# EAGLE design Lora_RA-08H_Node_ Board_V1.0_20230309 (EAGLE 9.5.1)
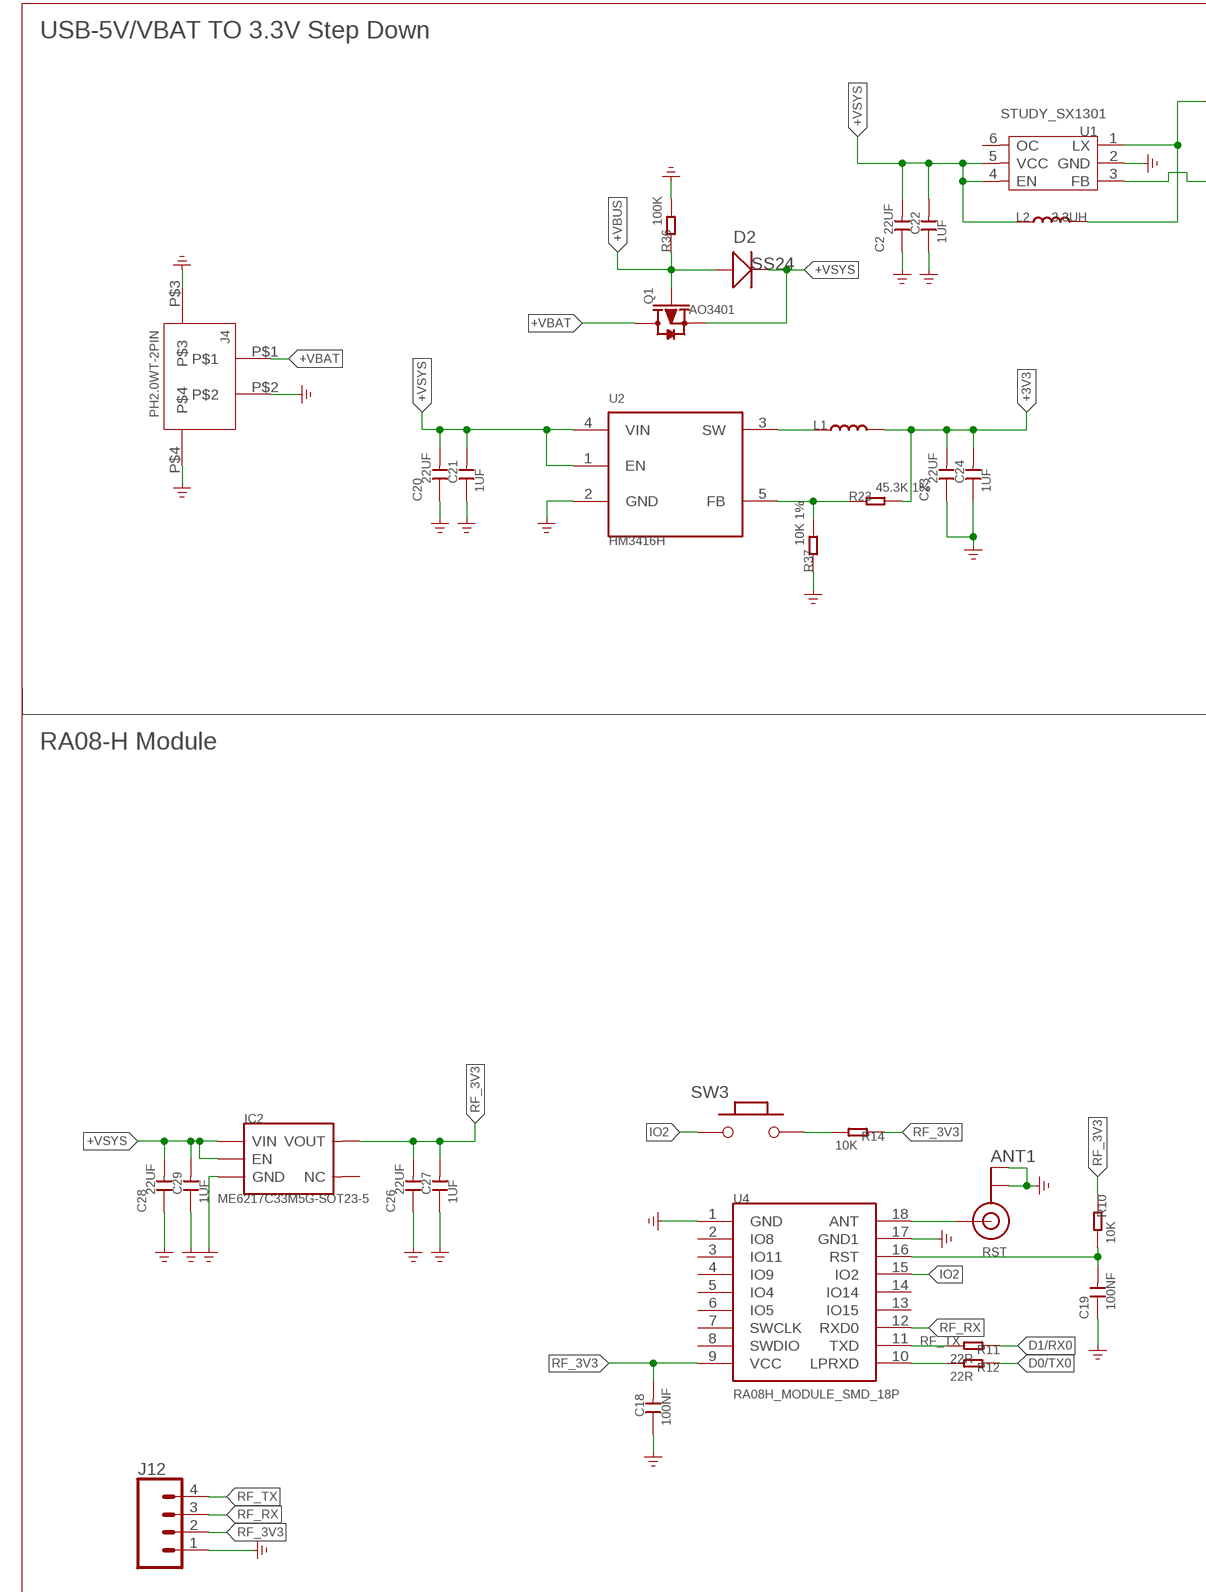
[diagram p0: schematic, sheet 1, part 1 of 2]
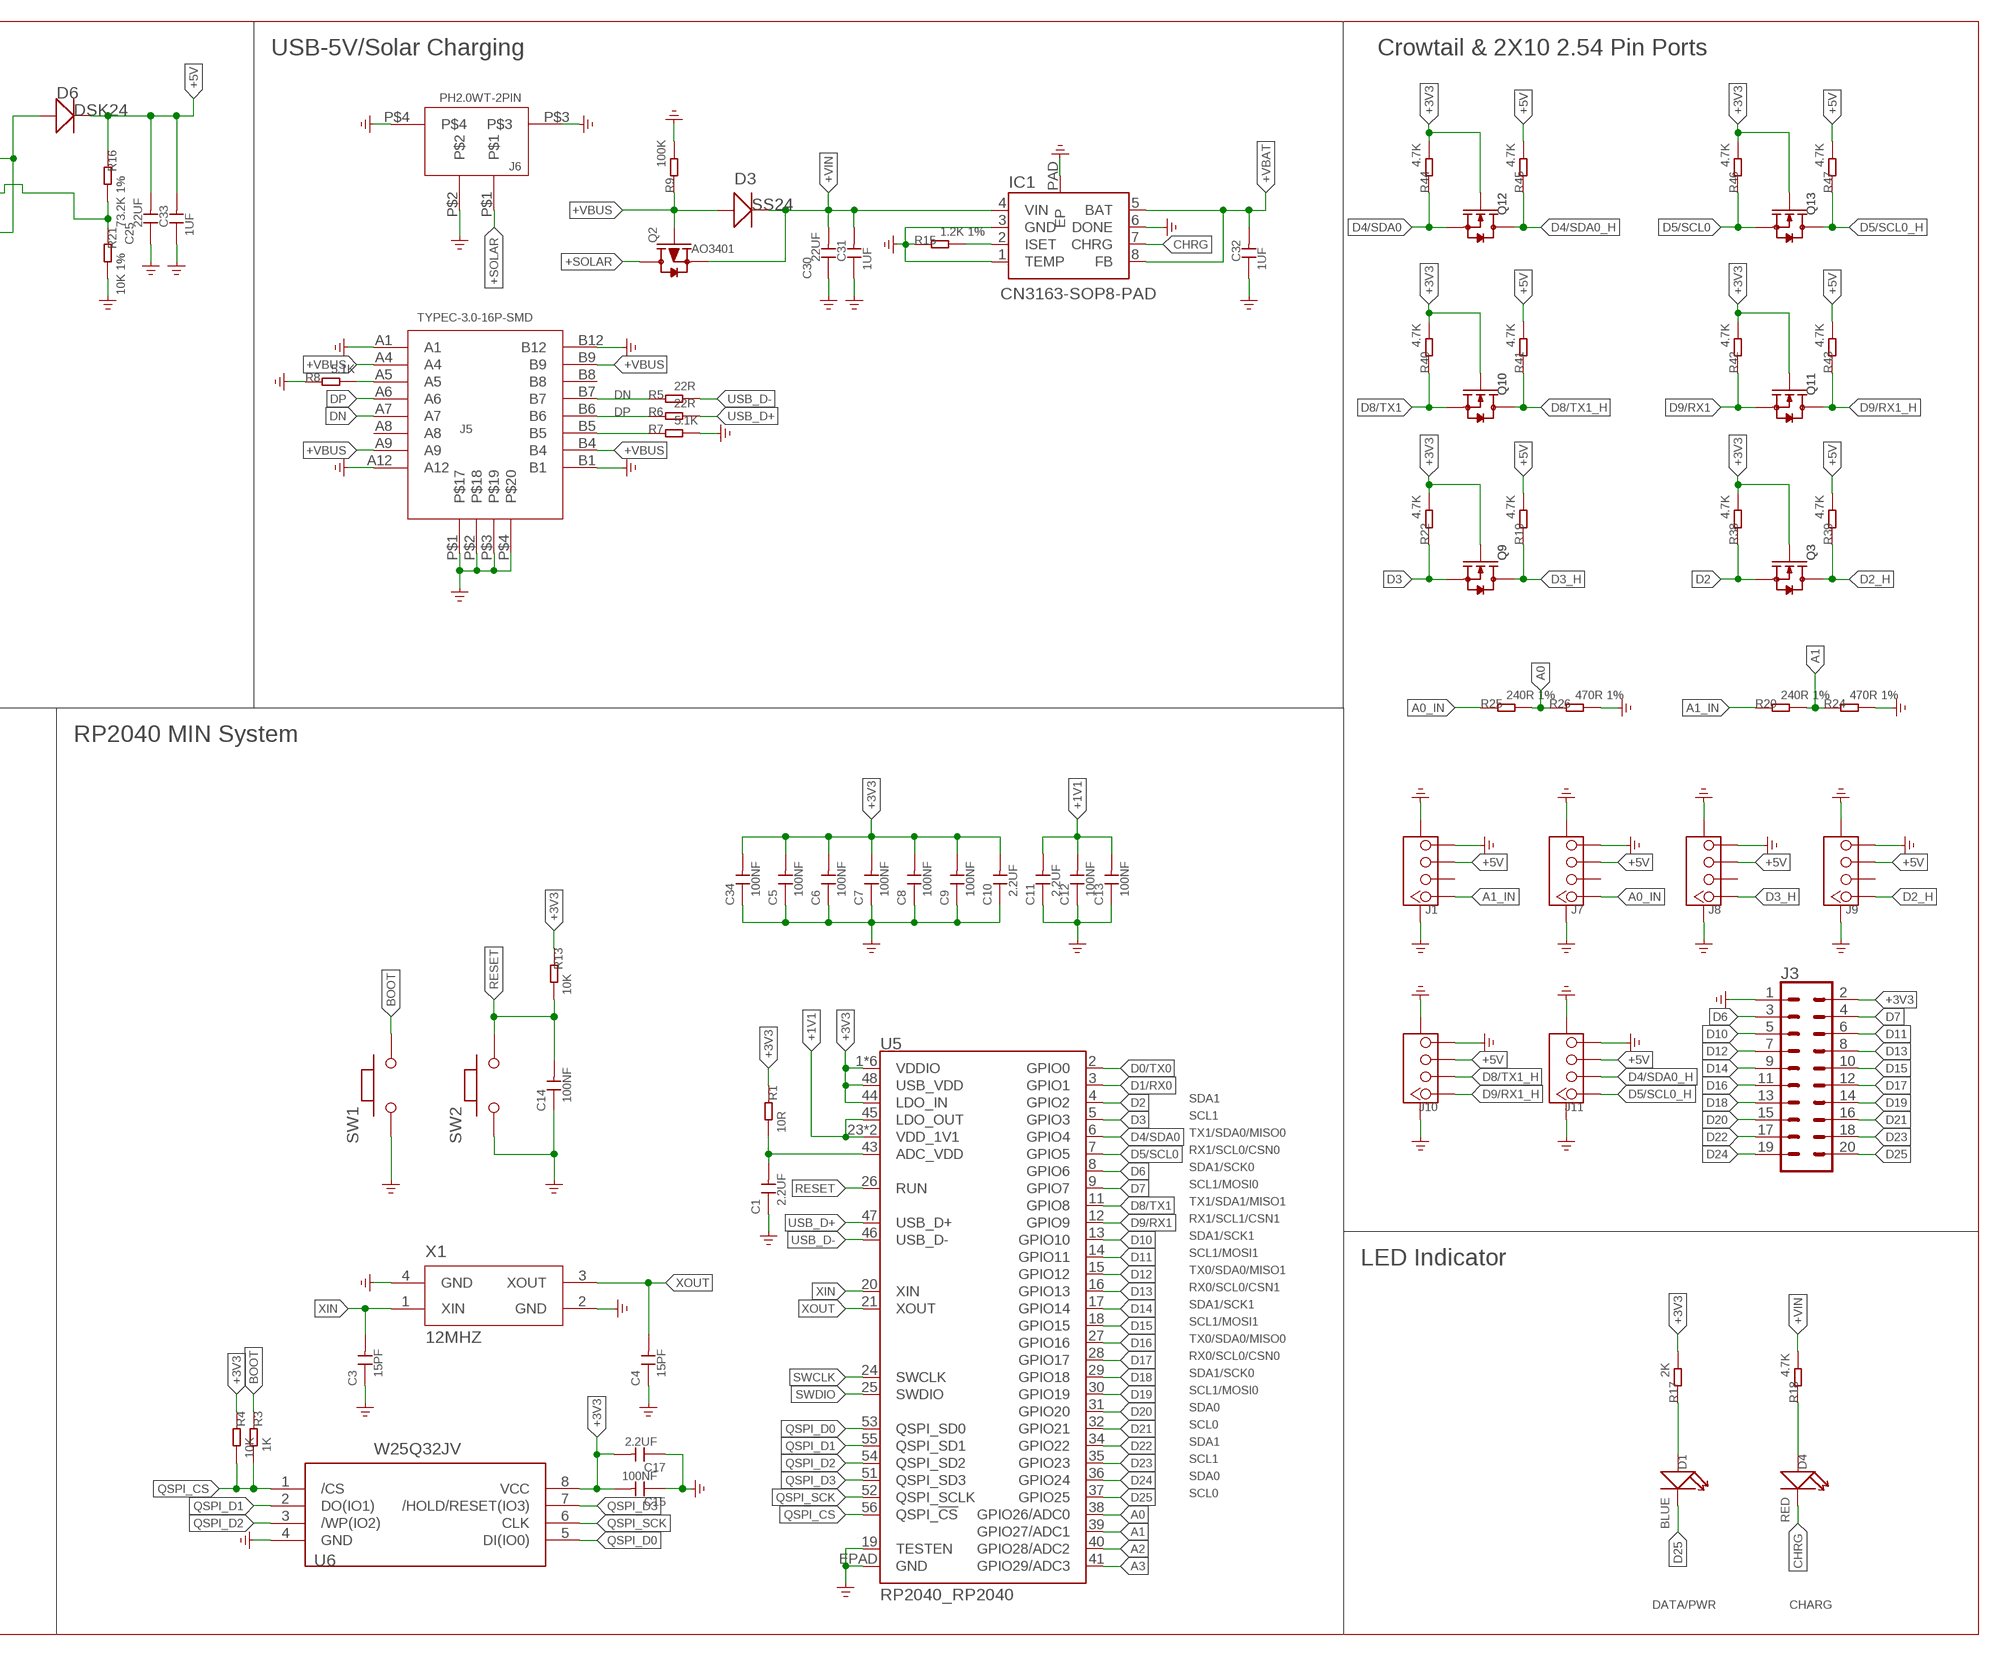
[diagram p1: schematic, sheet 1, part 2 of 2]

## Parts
ANT1  SPARKFUN2_U.FL  [SPARKFUN2_U.FL]
C1  2.2UF  CAPC0402-1  [0402]
C2  22UF  C0805  [C0805]
C3  15PF  CAPC0402-1  [0402]
C4  15PF  CAPC0402-1  [0402]
C5  100NF  CAPC0402-1  [0402]
C6  100NF  CAPC0402-1  [0402]
C7  100NF  CAPC0402-1  [0402]
C8  100NF  CAPC0402-1  [0402]
C9  100NF  CAPC0402-1  [0402]
C10  2.2UF  CAPC0402-1  [0402]
C11  2.2UF  CAPC0402-1  [0402]
C12  100NF  CAPC0402-1  [0402]
C13  100NF  CAPC0402-1  [0402]
C14  100NF  CAPC0402-1  [0402]
C15  100NF  CAPC0402-1  [0402]
C17  2.2UF  CAPC0402-1  [0402]
C18  100NF  C0603  [C0603]
C19  100NF  CAPC0402-1  [0402]
C20  22UF  C0805  [C0805]
C21  1UF  C0603  [C0603]
C22  1UF  C0603  [C0603]
C23  22UF  C0805  [C0805]
C24  1UF  C0603  [C0603]
C25  22UF  C0805  [C0805]
C26  22UF  C0805  [C0805]
C27  1UF  C0603  [C0603]
C28  22UF  C0805  [C0805]
C29  1UF  C0603  [C0603]
C30  22UF  C0805  [C0805]
C31  1UF  C0603  [C0603]
C32  1UF  C0603  [C0603]
C33  1UF  C0603  [C0603]
C34  100NF  CAPC0402-1  [0402]
D1  BLUE  LED-SMT0603  [LED0603]
D2  SS24  DIODEB130L-13-F  [SMA]
D3  SS24  DIODEB130L-13-F  [SMA]
D4  RED  LED-SMT0603  [LED0603]
D6  DSK24  DIODE  [D_SOD123FL]
IC1  CN3163-SOP8-PAD  [SOP8-PAD]
IC2  ME6217C33M5G-SOT23-5  [IC_SOT23-5]
J1  CONNECTOR_TWIG-4P-2.0-SMD-FEMALE-REINFORCE90D  [CONNECTOR_4P-SMD-2.0-90D]
J3  CONN_10X22X10-DSY-P2.54  [2X10-DSY-P2.54]
J4  PH2.0WT-2PIN  [PH2.0WT-2PIN]
J5  TYPEC-3.0-16P-SMD  [KEVIN_3.0TYPEC-SMD]
J6  PH2.0WT-2PIN  [PH2.0WT-2PIN]
J7  CONNECTOR_TWIG-4P-2.0-SMD-FEMALE-REINFORCE90D  [CONNECTOR_4P-SMD-2.0-90D]
J8  CONNECTOR_TWIG-4P-2.0-SMD-FEMALE-REINFORCE90D  [CONNECTOR_4P-SMD-2.0-90D]
J9  CONNECTOR_TWIG-4P-2.0-SMD-FEMALE-REINFORCE90D  [CONNECTOR_4P-SMD-2.0-90D]
J10  CONNECTOR_TWIG-4P-2.0-SMD-FEMALE-REINFORCE90D  [CONNECTOR_4P-SMD-2.0-90D]
J11  CONNECTOR_TWIG-4P-2.0-SMD-FEMALE-REINFORCE90D  [CONNECTOR_4P-SMD-2.0-90D]
J12  CONN_041.27MM  [1X04_1.27MM]
L1  LL0420  [L0420]
L2  3.3UH  LL0420  [L0420]
Q1  AO3401  MOSFET-PSOT23  [PMOS_SOT23]
Q2  AO3401  MOSFET-PSOT23  [PMOS_SOT23]
Q3  MOSFET-NSI1304BDL  [MOS_SOT323]
Q9  MOSFET-NSI1304BDL  [MOS_SOT323]
Q10  MOSFET-NSI1304BDL  [MOS_SOT323]
Q11  MOSFET-NSI1304BDL  [MOS_SOT323]
Q12  MOSFET-NSI1304BDL  [MOS_SOT323]
Q13  MOSFET-NSI1304BDL  [MOS_SOT323]
R1  10R  RES-0402  [R0402]
R3  1K  RES-0402  [R0402]
R4  10K  RES-0402  [R0402]
R5  22R  RES-0402  [R0402]
R6  22R  RES-0402  [R0402]
R7  5.1K  RES-0402  [R0402]
R8  5.1K  RES-0402  [R0402]
R9  100K  RES-0402  [R0402]
R10  10K  RES-0402  [R0402]
R11  22R  RES-0402  [R0402]
R12  22R  RES-0402  [R0402]
R13  10K  RES-0402  [R0402]
R14  10K  RES-0402  [R0402]
R15  1.2K 1%  RES-0402  [R0402]
R16  73.2K 1%  RES-0402  [R0402]
R17  2K  RES-0402  [R0402]
R18  4.7K  RES-0402  [R0402]
R19  4.7K  RES-0402  [R0402]
R20  240R 1%  RES-0402  [R0402]
R21  10K 1%  RES-0402  [R0402]
R22  4.7K  RES-0402  [R0402]
R23  45.3K 1%  RES-0402  [R0402]
R24  470R 1%  RES-0402  [R0402]
R25  240R 1%  RES-0402  [R0402]
R26  470R 1%  RES-0402  [R0402]
R36  100K  RES-0402  [R0402]
R37  10K 1%  RES-0402  [R0402]
R38  4.7K  RES-0402  [R0402]
R39  4.7K  RES-0402  [R0402]
R40  4.7K  RES-0402  [R0402]
R41  4.7K  RES-0402  [R0402]
R42  4.7K  RES-0402  [R0402]
R43  4.7K  RES-0402  [R0402]
R44  4.7K  RES-0402  [R0402]
R45  4.7K  RES-0402  [R0402]
R46  4.7K  RES-0402  [R0402]
R47  4.7K  RES-0402  [R0402]
SW1  MYSMD_PB157_4.3X3  [MYSMD_157SW]
SW2  MYSMD_PB157_4.3X3  [MYSMD_157SW]
SW3  MYSMD_PB157_4.3X3  [MYSMD_157SW]
U1  STUDY_SX1301  [STUDY_SOT23-6L]
U2  HM3416H  [IC_SOT23-5]
U4  RA08H_MODULE_SMD_18P  [RA08H_MODULE_SMT_18P]
U5  RP2040_RP2040  [RP2040_QFN-56]
U6  W25Q32JV  [SELF_SOIC-8-208MIL]
X1  12MHZ  XTAL-SMD3225  [SMD3225]

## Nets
+1V1: C11.2 C12.2 C13.2 U5.23(VDD_1V1) U5.45(LDO_OUT) U5.50(VDD_1V1)
+3V3: C5.2 C6.2 C7.2 C8.2 C9.2 C10.2 C15.2 C17.2 C23.2 C24.2 C34.2 J3.2 L1.2 Q3.1(G) Q9.1(G) Q10.1(G) Q11.1(G) Q12.1(G) Q13.1(G) R1.1 R4.1 R13.1 R17.2 R22.2 R23.2 R38.2 R40.2 R42.2 R44.2 R46.2 U5.1(VDDIO) U5.10(VDDIO) U5.22(VDDIO) U5.33(VDDIO) U5.42(VDDIO) U5.44(LDO_IN) U5.48(USB_VDD) U5.49(VDDIO) U6.8(VCC)
+5V: C25.2 C33.2 D6.- J1.3 J7.3 J8.3 J9.3 J10.3 J11.3 R16.1 R19.2 R39.2 R41.2 R43.2 R45.2 R47.2
+SOLAR: J6.P$1 Q2.3(D)
+VBAT: C32.2 IC1.5(BAT) IC1.8(FB) J4.P$1 Q1.3(D)
+VBUS: D2.2(+) D3.2(+) J5.A4 J5.A9 J5.B4 J5.B9 Q1.1(G) Q2.1(G) R9.1 R36.1
+VIN: C30.2 C31.2 D3.1(-) IC1.4(VIN) Q2.2(S) R18.2
+VSYS: C2.2 C20.2 C21.2 C22.2 C28.2 C29.2 D2.1(-) IC2.1(VIN) IC2.3(EN) L2.1 Q1.2(S) U1.4(EN) U1.5(VCC) U2.1(EN) U2.4(VIN)
A0: R25.2 R26.1 U5.38(GPIO26/ADC0)
A0_IN: J7.1 R25.1
A1: R20.2 R24.1 U5.39(GPIO27/ADC1)
A1_IN: J1.1 R20.1
A2: U5.40(GPIO28/ADC2)
A3: U5.41(GPIO29/ADC3)
BOOT: R3.1 SW1.2
CHRG: D4.- IC1.7(CHRG)
D0/TX0: R12.1 U5.2(GPIO0)
D1/RX0: R11.1 U5.3(GPIO1)
D2: Q3.2(S) R38.1 U5.4(GPIO2)
D2_H: J9.1 Q3.3(D) R39.1
D3: Q9.2(S) R22.1 U5.5(GPIO3)
D3_H: J8.1 Q9.3(D) R19.1
D4/SDA0: Q12.2(S) R44.1 U5.6(GPIO4)
D4/SDA0_H: J11.2 Q12.3(D) R45.1
D5/SCL0: Q13.2(S) R46.1 U5.7(GPIO5)
D5/SCL0_H: J11.1 Q13.3(D) R47.1
D6: J3.3 U5.8(GPIO6)
D7: J3.4 U5.9(GPIO7)
D8/TX1: Q10.2(S) R40.1 U5.11(GPIO8)
D8/TX1_H: J10.2 Q10.3(D) R41.1
D9/RX1: Q11.2(S) R42.1 U5.12(GPIO9)
D9/RX1_H: J10.1 Q11.3(D) R43.1
D10: J3.5 U5.13(GPIO10)
D11: J3.6 U5.14(GPIO11)
D12: J3.7 U5.15(GPIO12)
D13: J3.8 U5.16(GPIO13)
D14: J3.9 U5.17(GPIO14)
D15: J3.10 U5.18(GPIO15)
D16: J3.11 U5.27(GPIO16)
D17: J3.12 U5.28(GPIO17)
D18: J3.13 U5.29(GPIO18)
D19: J3.14 U5.30(GPIO19)
D20: J3.15 U5.31(GPIO20)
D21: J3.16 U5.32(GPIO21)
D22: J3.17 U5.34(GPIO22)
D23: J3.18 U5.35(GPIO23)
D24: J3.19 U5.36(GPIO24)
D25: D1.- J3.20 U5.37(GPIO25)
DN: J5.A7 J5.B7 R5.1
DP: J5.A6 J5.B6 R6.1
GND: ANT1.P$1(GND) ANT1.P$2(GND) C1.1 C2.1 C3.1 C4.1 C5.1 C6.1 C7.1 C8.1 C9.1 C10.1 C11.1 C12.1 C13.1 C14.1 C15.1 C17.1 C18.1 C19.1 C20.1 C21.1 C22.1 C23.1 C24.1 C25.1 C26.1 C27.1 C28.1 C29.1 C30.1 C31.1 C32.1 C33.1 C34.1 IC1.1(TEMP) IC1.3(GND) IC1.6(DONE) IC1.PAD(EP) IC2.2(GND) J1.4 J1.SS1 J1.SS2 J3.1 J4.P$2 J4.P$3 J4.P$4 J5.A1 J5.A12 J5.B1 J5.B12 J5.P$1 J5.P$2 J5.P$3 J5.P$4 J6.P$2 J6.P$3 J6.P$4 J7.4 J7.SS1 J7.SS2 J8.4 J8.SS1 J8.SS2 J9.4 J9.SS1 J9.SS2 J10.4 J10.SS1 J10.SS2 J11.4 J11.SS1 J11.SS2 J12.1 R7.2 R8.1 R9.2 R15.1 R21.2 R24.2 R26.2 R36.2 R37.1 SW1.1 SW2.1 U1.2(GND) U2.2(GND) U4.1(GND) U4.17(GND1) U5.19(TESTEN) U5.EPAD(GND) U6.4(GND) X1.2(GND) X1.4(GND)
IO2: SW3.1 U4.15(IO2)
N$1: C1.2 R1.2 U5.43(ADC_VDD)
N$2: J5.B5 R7.1
N$3: L1.1 U2.3(SW)
N$4: D6.+ L2.2 U1.1(LX)
N$5: R12.2 U4.10(LPRXD)
N$6: J5.A5 R8.2
N$7: R14.2 SW3.2
N$8: ANT1.P$3(SIGNAL) U4.18(ANT)
N$9: R23.1 R37.2 U2.5(FB)
N$10: IC1.2(ISET) R15.2
N$11: D4.+ R18.1
N$13: R16.2 R21.1 U1.3(FB)
N$14: D1.+ R17.1
QSPI_CS: R3.2 R4.2 U5.56(QSPI_!CS!) U6.1(/CS)
QSPI_D0: U5.53(QSPI_SD0) U6.5(DI(IO0))
QSPI_D1: U5.55(QSPI_SD1) U6.2(DO(IO1))
QSPI_D2: U5.54(QSPI_SD2) U6.3(/WP(IO2))
QSPI_D3: U5.51(QSPI_SD3) U6.7(/HOLD/RESET(IO3))
QSPI_SCK: U5.52(QSPI_SCLK) U6.6(CLK)
RESET: C14.2 R13.2 SW2.2 U5.26(RUN)
RF_3V3: C18.2 C26.2 C27.2 IC2.5(VOUT) J12.2 R10.1 R14.1 U4.9(VCC)
RF_RX: J12.3 U4.12(RXD0)
RF_TX: J12.4 R11.2 U4.11(TXD)
RST: C19.2 R10.2 U4.16(RST)
SWCLK: U5.24(SWCLK)
SWDIO: U5.25(SWDIO)
USB_D+: R6.2 U5.47(USB_D+)
USB_D-: R5.2 U5.46(USB_D-)
XIN: C3.2 U5.20(XIN) X1.1(XIN)
XOUT: C4.2 U5.21(XOUT) X1.3(XOUT)
Unconnected: IC2.4(NC) J1.2 J5.A8 J5.B8 J7.2 J8.2 J9.2 U1.6(OC) U4.2(IO8) U4.3(IO11) U4.4(IO9) U4.5(IO4) U4.6(IO5) U4.7(SWCLK) U4.8(SWDIO) U4.13(IO15) U4.14(IO14)

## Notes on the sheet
- USB-5V/VBAT TO 3.3V Step Down | USB-5V/Solar Charging | Crowtail & 2X10 2.54 Pin Ports
- RA08-H Module | RP2040 MIN System
- SDA1
- SCL1
- TX1/SDA0/MISO0
- RX1/SCL0/CSN0
- SDA1/SCK0
- SCL1/MOSI0
- TX1/SDA1/MISO1
- RX1/SCL1/CSN1
- SDA1/SCK1
- SCL1/MOSI1
- LED Indicator
- TX0/SDA0/MISO1
- RX0/SCL0/CSN1
- SDA1/SCK1
- SCL1/MOSI1
- TX0/SDA0/MISO0
- RX0/SCL0/CSN0
- SDA1/SCK0
- SCL1/MOSI0
- SDA0
- SCL0
- SDA1
- SCL1
- SDA0
- SCL0
- DATA/PWR | CHARG

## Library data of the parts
ANT1 = Lora_RA-08H_Node_ Board:SPARKFUN2_U.FL
C1 C3-C15 C17 C19 C34 = Lora_RA-08H_Node_ Board:CAP*
C2 C20 C23 C25 C26 C28 C30 = Lora_RA-08H_Node_ Board:C0805
C18 C21 C22 C24 C27 C29 C31-C33 = Lora_RA-08H_Node_ Board:C0603
D1 D4 = Lora_RA-08H_Node_ Board:LED-SMT*
D2 D3 D6 = Lora_RA-08H_Node_ Board:DIODE*
IC1 = Lora_RA-08H_Node_ Board:CN3163-SOP8-PAD
IC2 = Lora_RA-08H_Node_ Board:ME6217C33M5G-SOT23-5
J1 J7-J11 = Lora_RA-08H_Node_ Board:CONNECTOR_TWIG-4P-2.0-SMD-FEMALE-REINFORCE
J3 = Lora_RA-08H_Node_ Board:CONN_10X2: Multi connection point. Often used as Generic Header-pin footprint for 0.1 inch spaced/style header connections On any of the 0.1 inch spaced packages, you can populate with these: Break Away Headers - Straight (PRT-00116) Break Away Male Headers - Right Angle (PRT-00553) Female Headers (PRT-00115)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
J4 J6 = Lora_RA-08H_Node_ Board:PH2.0WT-2PIN
J5 = Lora_RA-08H_Node_ Board:TYPEC-3.0-16P-SMD
J12 = Lora_RA-08H_Node_ Board:CONN_04: Multi connection point. Often used as Generic Header-pin footprint for 0.1 inch spaced/style header connections On any of the 0.1 inch spaced packages, you can populate with these: Break Away Headers - Straight (PRT-00116) Break Away Male Headers - Right Angle (PRT-00553) Female Headers (PRT-00115)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
L1 L2 = Lora_RA-08H_Node_ Board:L*
Q1 Q2 = Lora_RA-08H_Node_ Board:MOSFET-P: IRLL014: http://www.vishay.com/docs/91319/sihll014.pdf
Q3 Q9-Q13 = Lora_RA-08H_Node_ Board:MOSFET-N*: IRLL014: http://www.vishay.com/docs/91319/sihll014.pdf
R1 R3-R26 R36-R47 = Lora_RA-08H_Node_ Board:RES*
SW1-SW3 = Lora_RA-08H_Node_ Board:MYSMD_PB157_4.3X3
U1 = Crowtail- Air Quality Sensor  v1.0:STUDY_SX1301
U2 = Lora_RA-08H_Node_ Board:HM3416H
U4 = Lora_RA-08H_Node_ Board:RA08H_MODULE_SMD_18P
U5 = Lora_RA-08H_Node_ Board:RP2040_RP2040: Raspberry Pi RP2040 MCU 56-pin 32-bit Microcontroller with 264kB of SRAM and external flash support up to 16MB Getting Started with the RP2040 Dual-core ARM Cortex M0+ processor, flexible clock running up to 133 MHz 264kB of SRAM, and QSPI control of common flash memory USB 1.1 Host and Device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; PROD_ID: IC-15502
U6 = Lora_RA-08H_Node_ Board:W25Q32JV
X1 = Lora_RA-08H_Node_ Board:XTAL-SMD3225

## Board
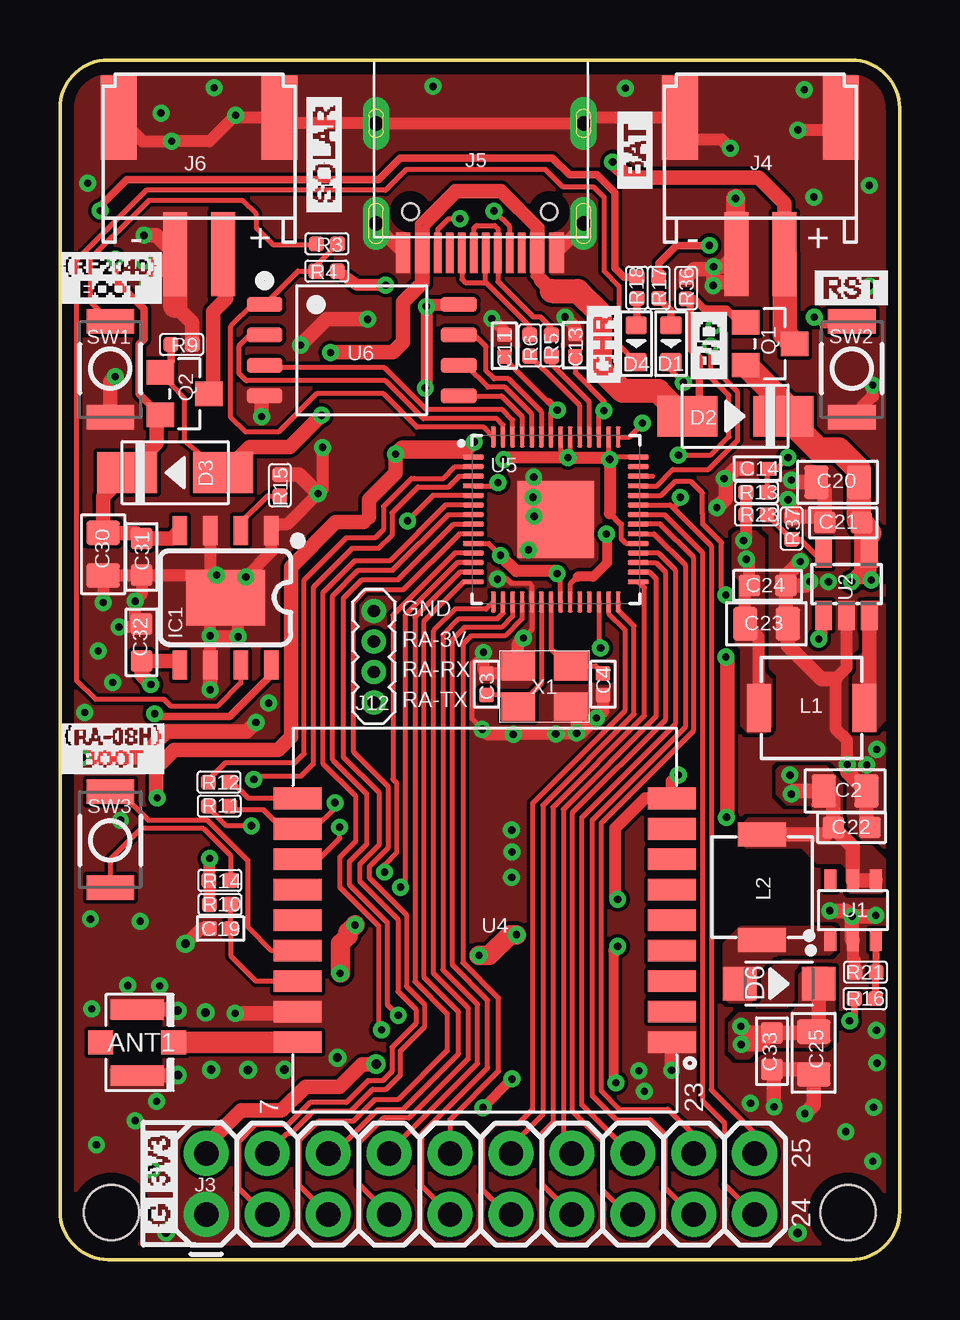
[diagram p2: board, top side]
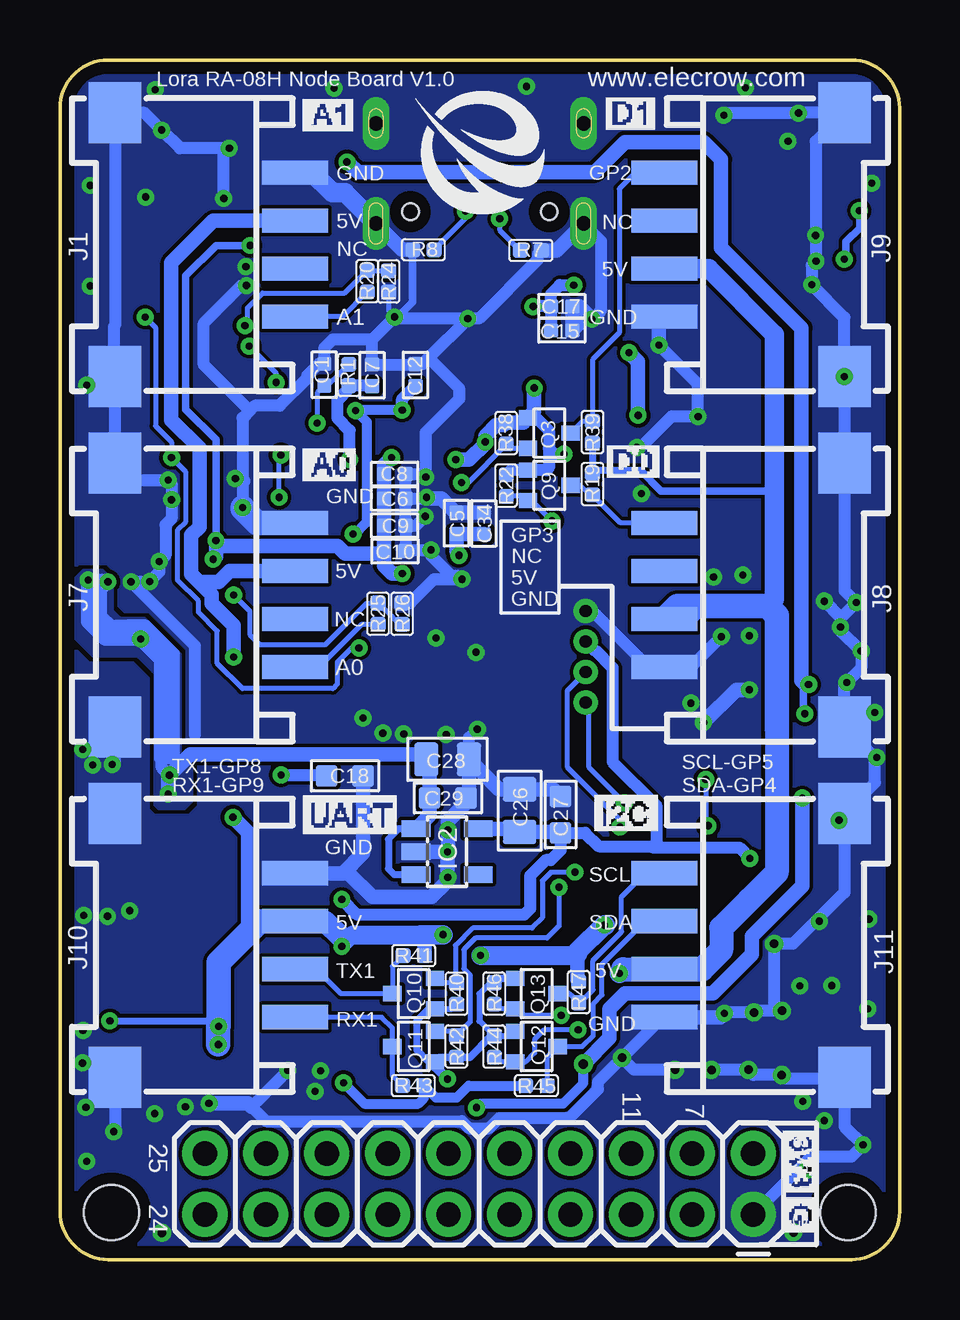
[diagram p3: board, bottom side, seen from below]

Size 35 x 50 mm. Coordinates in mm from the lower left corner, seen from the top.
Outline: 0,2 0,48 arc-90 2,50 33,50 arc-90 35,48 35,2 arc-90 33,0 2,0 arc-90 0,2
Copper layers (1*16): Top 0.035mm / dielectric 1.5mm / Bottom 0.035mm
Design rules "default *": minimum track width 8mil, minimum drill 0.3mm, track to track 6mil, track to pad 6mil, pad to pad 6mil, via to via 6mil, smd to smd 6mil, copper to edge 20mil, drill to drill 6mil, minimum pad ring 10mil, minimum via ring 8mil, stop-mask expansion 4mil, vias tented up to drill 100mil, thermal gap 10mil
Holes 2.3 mm at 2.15,1.95 32.85,1.95
tRestrict: 19 lines

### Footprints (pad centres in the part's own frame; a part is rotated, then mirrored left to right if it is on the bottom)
SPARKFUN2_U.FL = smd 2.2 x 0.85: P$1 0,1.375; P$2 0,-1.375 | smd 1.05 x 1: P$3 1.525,0; P$4 -1.525,0
0402 = smd 0.6 x 0.6: 1 -0.45,0; 2 0.45,0
C0805 = smd 1.016 x 1.397: 1 -0.889,0; 2 0.889,0
C0603 = smd 0.889 x 0.889: 1 -0.762,0; 2 0.762,0
LED0603 = smd 0.762 x 0.889: + -0.762,0; - 0.762,0
SMA = smd 2.5 x 1.7: 1 2,0; 2 -2,0
D_SOD123FL = smd 1.397 x 1.397: + -1.651,0; - 1.651,0
SOP8-PAD = smd 0.6 x 1.2: 1 -1.905,-2.8; 2 -0.635,-2.8; 3 0.635,-2.8; 4 1.905,-2.8; 5 1.905,2.8; 6 0.635,2.8; 7 -0.635,2.8; 8 -1.905,2.8 | smd 3.3 x 2.311: PAD 0,0
IC_SOT23-5 = smd 0.69 x 1.2: 1 -0.95,-1.3; 2 0,-1.3; 3 0.95,-1.3; 4 0.95,1.3; 5 -0.95,1.3
CONNECTOR_4P-SMD-2.0-90D = smd 1.01 x 2.74: 1 -3,-0.1; 2 -1,-0.1; 3 1,-0.1; 4 3,-0.1 | smd 2.54 x 2.184: SS1 -5.5,7.4; SS2 5.5,7.4
2X10-DSY-P2.54 = drill 1.016 pad 1.88: 1 0,0; 2 0,2.54; 3 2.54,0; 4 2.54,2.54; 5 5.08,0; 6 5.08,2.54; 7 7.62,0; 8 7.62,2.54; 9 10.16,0; 10 10.16,2.54; 11 12.7,0; 12 12.7,2.54; 13 15.24,0; 14 15.24,2.54; 15 17.78,0; 16 17.78,2.54; 17 20.32,0; 18 20.32,2.54; 19 22.86,0; 20 22.86,2.54
PH2.0WT-2PIN = smd 1 x 3.5: P$1 -1,0; P$2 1,0 | smd 1.5 x 3.5: P$3 -3.35,-5.7; P$4 3.35,-5.7
KEVIN_3.0TYPEC-SMD = smd 0.3 x 1.7: A1 -3.35,0.5; A4 -2.55,0.5; A5 -1.25,0.5; A6 -0.25,0.5; A7 0.25,0.5; A8 1.25,0.5; A9 2.55,0.5; A12 3.35,0.5; B1 3.05,0.5; B4 2.25,0.5; B5 1.75,0.5; B6 0.75,0.5; B7 -0.75,0.5; B8 -1.75,0.5; B9 -2.25,0.5; B12 -3.05,0.5 | drill 0.6 pad 1.016 long: P$1 -4.325,-0.72; P$2 4.325,-0.72; P$3 -4.325,-4.9; P$4 4.325,-4.9 | hole 0.68: -2.89,-1.22; 2.89,-1.22
1X04_1.27MM = drill 0.508 pad 1: 1 0,0; 2 1.27,0; 3 2.54,0; 4 3.81,0
L0420 = smd 2 x 1: 1 0,2.2; 2 0,-2.2
PMOS_SOT23 = smd 1.016 x 1.143: 1 -0.889,-1.016; 2 0.889,-1.016; 3 0,1.016
MOS_SOT323 = smd 0.635 x 0.762: 1 -0.635,-0.889; 2 0.635,-0.889; 3 0,0.889
R0402 = smd 0.635 x 0.635: 1 -0.445,0; 2 0.445,0
MYSMD_157SW = smd 1.016 x 1.981: 1 0,0; 2 4,0
STUDY_SOT23-6L = smd 0.5 x 0.9: 1 -0.961,-1.212; 2 -0.011,-1.212; 3 0.94,-1.212; 4 0.94,1.288; 5 -0.011,1.288; 6 -0.961,1.288
RA08H_MODULE_SMT_18P = smd 2 x 0.9: 1 -7.8,5.08; 2 -7.8,3.81; 3 -7.8,2.54; 4 -7.8,1.27; 5 -7.8,0; 6 -7.8,-1.27; 7 -7.8,-2.54; 8 -7.8,-3.81; 9 -7.8,-5.08; 10 7.8,-5.08; 11 7.8,-3.81; 12 7.8,-2.54; 13 7.8,-1.27; 14 7.8,0; 15 7.8,1.27; 16 7.8,2.54; 17 7.8,3.81; 18 7.8,5.08
RP2040_QFN-56 = smd 0.875 x 0.2: 1 -3.437,2.6; 2 -3.437,2.2; 3 -3.437,1.8; 4 -3.437,1.4; 5 -3.437,1; 6 -3.437,0.6; 7 -3.437,0.2; 8 -3.437,-0.2; 9 -3.437,-0.6; 10 -3.437,-1; 11 -3.437,-1.4; 12 -3.437,-1.8; 13 -3.437,-2.2; 14 -3.437,-2.6; 29 3.437,-2.6; 30 3.437,-2.2; 31 3.437,-1.8; 32 3.437,-1.4; 33 3.437,-1; 34 3.437,-0.6; 35 3.437,-0.2; 36 3.437,0.2; 37 3.437,0.6; 38 3.437,1; 39 3.437,1.4; 40 3.437,1.8; 41 3.437,2.2; 42 3.437,2.6 | smd 0.2 x 0.875: 15 -2.6,-3.437; 16 -2.2,-3.437; 17 -1.8,-3.437; 18 -1.4,-3.437; 19 -1,-3.437; 20 -0.6,-3.437; 21 -0.2,-3.437; 22 0.2,-3.437; 23 0.6,-3.437; 24 1,-3.437; 25 1.4,-3.437; 26 1.8,-3.437; 27 2.2,-3.437; 28 2.6,-3.437; 43 2.6,3.437; 44 2.2,3.437; 45 1.8,3.437; 46 1.4,3.437; 47 1,3.437; 48 0.6,3.437; 49 0.2,3.437; 50 -0.2,3.437; 51 -0.6,3.437; 52 -1,3.437; 53 -1.4,3.437; 54 -1.8,3.437; 55 -2.2,3.437; 56 -2.6,3.437 | smd 3.2 x 3.2: EPAD 0,0
SELF_SOIC-8-208MIL = smd 1.5 x 0.635: 1 -4.05,1.905; 2 -4.05,0.635; 3 -4.05,-0.635; 4 -4.05,-1.905; 5 4.05,-1.905; 6 4.05,-0.635; 7 4.05,0.635; 8 4.05,1.905
SMD3225 = smd 1.4 x 1.2: 1 -1.1,-0.85; 2 1.1,-0.85; 3 1.1,0.85; 4 -1.1,0.85

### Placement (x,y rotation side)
ANT1  3.22,9.05 0 top
C1  23.98,36.88 270 bottom
C2  32.73,19.53 180 top
C3  17.78,23.98 270 top
C4  22.64,23.98 90 top
C5  18.47,30.69 270 bottom
C6  21.05,31.72 180 bottom
C7  21.99,36.86 270 bottom
C8  21.05,32.74 180 bottom
C9  21.05,30.59 180 bottom
C10  21.04,29.53 180 bottom
C11  18.53,38.09 270 top
C12  20.18,36.87 270 bottom
C13  21.48,38.11 270 top
C14  29.08,32.96 0 top
C15  14.08,38.73 180 bottom
C17  14.08,39.73 180 bottom
C18  23.12,20.16 180 bottom
C19  6.69,13.8 0 top
C20  32.42,32.4 0 top
C21  32.65,30.71 0 top
C22  33,18.01 180 top
C23  29.45,26.5 180 top
C24  29.5,28.1 180 top
C25  31.42,8.61 90 top
C26  15.84,18.71 270 bottom
C27  14.13,18.55 270 bottom
C28  18.84,20.85 180 bottom
C29  18.83,19.24 180 bottom
C30  1.8,29.4 90 top
C31  3.4,29.29 90 top
C32  3.4,25.72 270 top
C33  29.68,8.68 90 top
C34  17.33,30.68 270 bottom
D1  25.47,38.17 270 top
D2  28.15,35.15 0 top
D3  4.8,32.8 180 top
D4  24.02,38.17 270 top
D6  29.98,11.5 0 top
IC1  6.9,27.58 180 top
IC2  18.86,17 270 bottom
J1  25.3,42.3 90 bottom
J3  6.1,1.88 0 top
J4  29.2,41.9 180 top
J5  17.5,42.46 180 top
J6  5.8,41.9 180 top
J7  25.3,27.7 90 bottom
J8  9.7,27.7 270 bottom
J9  9.7,42.3 270 bottom
J10  25.3,13.1 90 bottom
J11  9.7,13.1 270 bottom
J12  13.08,27.03 270 top
L1  31.33,22.99 270 top
L2  29.27,15.52 0 top
Q1  29.6,38.17 270 top
Q2  5.2,36.09 270 top
Q3  14.6,34.45 270 bottom
Q9  14.6,32.27 270 bottom
Q10  20.25,11.09 90 bottom
Q11  20.25,8.88 90 bottom
Q12  15.13,8.88 270 bottom
Q13  15.13,11.09 270 bottom
R1  22.96,36.87 90 bottom
R3  11.13,42.34 0 top
R4  11.12,41.2 180 top
R5  20.49,38.1 270 top
R6  19.59,38.1 270 top
R7  15.37,42.06 0 bottom
R8  19.85,42.09 0 bottom
R9  5.07,38.14 0 top
R10  6.67,14.8 0 top
R11  6.64,18.9 0 top
R12  6.63,19.9 0 top
R13  29.04,31.98 0 top
R14  6.66,15.8 0 top
R15  9.17,32.27 270 top
R16  33.56,10.87 0 top
R17  24.96,40.5 90 top
R18  24.05,40.5 90 top
R19  12.8,32.32 90 bottom
R20  22.19,40.78 90 bottom
R21  33.58,11.98 180 top
R22  16.4,32.26 90 bottom
R23  29.04,31.04 180 top
R24  21.3,40.77 270 bottom
R25  21.74,26.92 90 bottom
R26  20.74,26.92 90 bottom
R36  26.1,40.49 90 top
R37  30.5,30.47 270 top
R38  16.4,34.45 90 bottom
R39  12.8,34.49 270 bottom
R40  18.47,11.09 270 bottom
R41  20.25,12.67 0 bottom
R42  18.48,8.88 270 bottom
R43  20.28,7.25 0 bottom
R44  16.9,8.88 90 bottom
R45  15.13,7.25 180 bottom
R46  16.9,11.09 90 bottom
R47  13.37,11.14 90 bottom
SW1  2.1,35.1 90 top
SW2  33.01,35.1 90 top
SW3  2.1,19.5 270 top
U1  33.07,14.52 0 top
U2  32.79,28.15 0 top
U4  17.71,14.14 180 top
U5  20.67,30.85 0 top
U6  12.58,37.9 0 top
U$55  [ELECROW-NEW]  20.23,43.56 0 bottom
X1  20.2,23.89 0 top

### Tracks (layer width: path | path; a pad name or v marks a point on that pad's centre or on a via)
+1V1  (via drill 0.3 pad 0.6)
  Top 0.203: 20.27,35.82 20.62,35.47 20.47,35.31 20.47,35.19 | 20.27,35.82 18.53,37.56 C11.2 | C13.2 21.48,36.97 22.68,35.77 v22.68,35.39 22.47,35.18 U5.45 | 20.73,35.45 v20.73,35.41 | U5.50 20.47,35.19 | 21.58,28.46 21.27,28.15 U5.23 | 20.47,35.19 20.73,35.45 | 20.27,35.82 20.36,35.82 20.73,35.45
  Top 0.406: v22.78,30.24 22.81,30.21 22.81,29.04 22.23,28.46 21.58,28.46
  Bottom 0.406: v20.73,35.41 20.75,35.43 22.64,35.43 v22.68,35.39 22.21,34.92 22.21,30.73 22.71,30.24 v22.78,30.24
  Bottom 0.508: v20.73,35.41 20.73,35.87 C12.2
+3V3  (via drill 0.3 pad 0.6, 0.4 pad 0.6)
  Top 0.203: U5.49 20.87,33.74 v21.18,33.43 21.27,33.52 U5.48 | U5.44 22.87,33.4 v22.92,33.35 23.01,33.44 U5.42 | 23.39,30.64 23.39,30.06 23.6,29.85 U5.33 | U5.10 17.87,29.85 v18.37,29.35 | U5.1 14.1,33.46 v13.99,33.57 | U5.22 20.87,28.45 v20.73,28.59
  Top 0.25: 22.92,31.11 23.39,30.64
  Top 0.305: R17.2 24.96,41.54 25.69,42.27 v27.07,42.27
  Top 0.406: v18.85,7.52 18.83,7.52 v17.64,6.33
  Top 0.508: 22.87,33.4 22.84,33.43 v21.18,33.43 18.59,33.43 v18.5,33.34 | v22.92,33.35 22.92,31.11 | U6.8 15.35,39.8 v15.27,39.73 15.27,36.37 v15.23,36.33 | v13.58,40.62 12.39,40.62 R4.1 | L1.2 29.13,25.93 C23.2 28.56,27.92 C24.2 28.74,29.07 v28.62,29.19 | v28.5,29.97 28.6,30.07 R23.2 R13.1 | v20.73,28.59 20.63,28.69 19.03,28.69 v18.37,29.35
  Top 0.6: v13.99,33.57 13.99,32.78 12.88,31.67 12.88,30.95 12.66,30.73 11.49,30.73 9.63,28.87 9.63,21.79 9.09,21.25 4.77,21.25 4.01,20.49 4.01,19.28 v4.05,19.24 | v13.18,8.14 12.59,8.14 11.65,7.2 10.23,7.2 9.24,6.21 9.16,6.21 7.55,6.21 6.39,5.05 6.1,4.76 J3.2
  Top 0.61: v17.27,34.08 17.03,33.84 14.26,33.84 v13.99,33.57
  Bottom 0.26: R46.2 17.06,11.53 17.52,11.07 17.52,9.94 R44.2 | R44.2 16.21,9.32 Q12.1 | 17.02,9.32 R44.2 | Q10.1 18.66,10.45 R40.2
  Bottom 0.3: Q11.1 19.64,8.24 20.12,8.73 20.12,9.96 19.63,10.45 Q10.1
  Bottom 0.305: v28.5,29.97 28.5,34.18 29.75,35.43 29.75,41.01 28.49,42.27 v27.07,42.27 | Q13.1 16.71,11.72 R46.2 | Q11.1 19.18,8.44 R42.2 17.91,8.44 17.03,9.32 R44.2
  Bottom 0.406: v17.64,6.33 17.46,6.51 14.02,6.51 13.18,7.35 v13.18,8.14 | v18.85,7.52 v18.85,7.53 19.37,8.04 Q11.1
  Bottom 0.508: C7.2 22.01,36.42 R1.1 22.96,36.28 23.44,35.8 23.44,35.08 22.92,34.56 v22.92,33.35 | C17.2 C15.2 | C17.2 15.06,39.73 v15.27,39.73 | C17.2 14.53,40.25 14.16,40.62 v13.58,40.62 | Q3.1 15.15,35.09 14.62,34.55 14.62,33.81 | 14.62,33.81 14.38,33.57 v13.99,33.57 | 14.62,33.81 14.62,32.99 14.71,32.91 Q9.1 16.2,32.91 R22.2
  Bottom 0.6: v4.05,19.24 v4.04,19.23 4.04,15.58 6.15,13.47 6.15,12.72 7.78,11.09 11.45,11.09 12.09,10.45 12.09,9.23 v13.18,8.14
  Bottom 0.61: v21.18,33.43 21.5,33.11 C8.2 C6.2 C9.2 C10.2 | v18.5,33.34 17.95,33.34 17.27,34.02 v17.27,34.08 17.27,34.32 16.81,34.78 16.51,34.78 R38.2 15.68,34.9 Q3.1 15.23,35.34 v15.23,36.33 | v28.62,29.19 28.5,29.31 v28.5,29.97 28.27,29.73 23.42,29.73 23.12,29.43 21.59,29.43 C10.2 | C34.2 C5.2 18.47,29.53 18.42,29.47 18.42,29.4 v18.37,29.35 | C10.2 21.49,28.93 21.15,28.59 v20.73,28.59
  pour Bottom (no thermals): 23.93,28.55 23.93,28.95 23.93,29.03
  pour Top (no thermals): 28.65,21.99 28.4,22.24 28.4,24.14 28.4,25.43 28.18,25.65 28.18,27.08 28.33,27.23 28.36,27.26 28.36,28.27 28.06,28.57 28.06,30.2 28.21,30.35 29.02,30.35 29.34,30.03 29.34,29.82 29.34,24.55 29.37,24.52 29.37,24.46 29.65,24.18 29.65,22.22 29.43,22 29.39,21.96 28.8,21.96 28.68,21.96
+5V  (via drill 0.3, 0.3 pad 0.6)
  Top 0.3: R16.1 33.12,10.15 v32.92,9.95
  Top 0.406: 11.7,11.95 v11.68,11.93 | v23.17,7.37 23.07,7.47 23.07,12.87 v23.25,13.05
  Top 0.6: D6.- 31.63,9.71 C25.2 31.36,9.44 C33.2 | C33.2 28.67,9.44 v28.39,9.72 | v27.76,25.11 27.82,25.05 27.82,18.46 v27.79,18.43 | C33.2 29.2,8.96 v28.4,8.96
  Top 0.813: v12.3,13.94 12.01,13.65 12.01,13.49 11.7,13.18 11.7,11.95 | v19.03,13.54 18.76,13.54 17.89,12.67 v17.46,12.67
  Bottom 0.3: 10.79,32.88 12.68,32.88 R19.2 R39.2 | v32.92,9.95 28.62,9.95 v28.39,9.72
  Bottom 0.305: 5.21,32.04 9.95,32.04 10.79,32.88
  Bottom 0.406: 10.03,12.1 J11.3 | v23.17,7.37 22.3,6.5 20.06,6.5 19.83,6.73 R43.2 19.34,6.76 18.45,6.76 17.96,7.25 R45.2
  Bottom 0.6: v23.25,13.05 22.76,13.54 | 19.97,13.54 19.81,13.38 R41.2 | 29.19,28.24 28.67,27.72 28.67,27.35 27.76,26.43 v27.76,25.11 | v27.79,18.43 27.16,17.8 27.16,13.62 | 13.43,12.75 13.43,11.65 R47.2
  Bottom 0.61: v23.25,13.05 23.25,13.41 | J7.3 27.92,28.7 28.38,28.24 29.19,28.24 29.53,28.58 29.53,30.19 29.18,30.54 29.18,33.82 30.36,35 30.36,41.55 28.61,43.3 J1.3
  Bottom 0.8: v17.46,12.67 13.5,12.67 | 22.76,13.54 19.97,13.54
  Bottom 0.813: J9.3 7.95,41.3 5.21,38.56 5.21,32.04 5.21,27.53 5.51,27.23 | 19.97,13.54 v19.03,13.54 | 13.5,12.67 13.43,12.75 13.43,12.83 12.31,13.95 v12.3,13.94 12.28,13.94 12.27,13.93 | 26.68,14.1 27.66,13.12 | v11.68,11.93 11.51,12.1
  Bottom 0.9: 23.25,13.41 23.94,14.1 J10.3
  Bottom 1: J8.3 9.03,26.7 8.49,27.24 | 11.51,12.1 10.03,12.1 | 8.23,12.1 7.43,12.9 7.43,13.83 6.27,14.99 6.26,14.99 5.12,16.13 5.12,22.12
  Bottom 1.016: 5.12,22.12 5.12,26.84 5.51,27.23 9.27,27.23 J8.3 | 10.03,12.1 8.23,12.1 | J10.3 26.68,14.1 27.16,13.62 | 27.22,13.56 27.66,13.12 28.39,12.39 v28.39,9.72 v28.4,9.71 v28.4,8.96
  pour Top (no thermals): 30.91,11.63 30.91,10.59 30.48,10.16 28.33,10.16 27.98,9.81 27.98,8.76 28.26,8.48 28.69,8.48 29.18,8.97 30.39,8.97 31.88,8.97 32.1,9.19 32.19,9.28 32.19,11.34 32.19,11.87 31.98,12.08 31.16,12.08 30.91,11.83 30.91,11.68
+SOLAR
  Top 0.6: J6.P$1 6.92,41.78 6.92,40.05 6.39,39.52 6.39,36.26 Q2.3
+VBAT  (via drill 0.3 pad 0.6)
  Top 0.305: IC1.8 8.8,24.36 7.08,22.63 4.07,22.63 v3.95,22.75
  Top 0.6: v3.79,23.97 3.4,24.36 C32.2 4.82,24.96 IC1.5
  Top 0.61: J4.P$1 30.2,44.03 29.14,45.09 23.7,45.09 v23.04,45.75
  Top 1.016: J4.P$1 30.21,38.58 Q1.3
  Bottom 0.305: v3.95,22.75 4.02,22.82 4.02,23.74 v3.79,23.97
  Bottom 0.61: v23.04,45.75 23,45.75 22.58,45.33 12.7,45.33 11.45,46.58 8.16,46.58 7.44,45.86 7.44,42.18 4.09,38.83 4.09,24.14 3.92,23.97 v3.79,23.97
+VBUS  (via drill 0.3 pad 0.6)
  Top 0.203: Q2.1 5.17,35.92 5.17,34.13 D3.2 | 28.55,39.06 Q1.1
  Top 0.3: J5.A4 20.05,40.82 20.05,40.7 19.75,41 J5.B9
  Top 0.305: 14.95,40.55 J5.A9 14.95,43.17 16.45,44.67 18.42,44.67 20.05,43.04 J5.A4 | 15.25,40.66 J5.B4 15.25,43.06 16.57,44.38 18.35,44.38 19.75,42.98 J5.B9 | R9.1 4.62,37.42 Q2.1 | D2.2 26.65,35.65 26.65,37.6 26.28,37.97 26.28,39.87 R36.1 26.43,40.05 26.86,39.62 27.79,39.62 28.34,39.06 28.55,39.06
  Top 0.6: 20.05,40.82 20.5,40.37
  Top 0.61: D3.2 6.83,32.8 7.9,33.87 9.58,33.87 v10.9,35.19 | v11.28,37.8 11.28,37.83 13.88,37.83 14.3,38.25 14.3,39.9 14.95,40.55
  Top 0.8: 25.98,35.15 D2.2
  Top 1: 25.98,35.15 24.93,36.2 23.45,36.2 22.51,37.14 22.51,39.44 21.58,40.37 20.5,40.37
  Bottom 0.61: v11.28,37.8 10.9,37.42 v10.9,35.19
+VIN  (via drill 0.3 pad 0.6)
  Top 0.305: v1.68,43.72 1.68,43.9 2.79,45.01 13.27,45.01 14.18,45.92 20.54,45.92 21.25,45.21 22.39,45.21 23.12,44.48 23.12,41.33 23.51,40.94 R18.2 | v2.3,41.7 v2.31,41.69 2.31,40.82 3.52,39.62 3.52,38.37 3.31,38.16 3.31,36.08 Q2.2
  Top 0.61: Q2.2 4.04,35.06 4.04,34.04 D3.1 1.8,31.8 C30.2 3.16,30.29 C31.2 4.67,30.05 IC1.4
  Bottom 0.305: v2.3,41.7 2.23,41.77 2.23,42.42 1.65,43 1.65,43.69 v1.68,43.72
+VSYS  (via drill 0.3 pad 0.6)
  Top 0.305: v31.63,25.86 31.84,26.07 U2.1
  Top 0.508: v33,28.25 33.15,28.4 33.74,28.4
  Top 0.6: v30.48,19.4 30.61,19.53 C2.2 32.24,19.13 C22.2 | C22.2 31.95,17.72 L2.1 | C22.2 33.06,17.19 U1.5 U1.4
  Top 0.61: 33.74,30.28 U2.4 33.74,28.4 v33.82,28.32 | C21.2 33.41,28.66 v33,28.25
  Top 1.016: 33.74,30.28 C21.2 33.31,30.81 C20.2 33.31,32.92 32.47,33.76 31.61,33.76 30.22,35.15 D2.1 30.15,35.72 Q1.2
  Bottom 0.3: 20.6,17.95 IC2.1 20.89,17.95 21.31,17.53 21.31,16.29 21.07,16.05 IC2.3
  Bottom 0.305: v31.63,25.86 31.66,25.89 31.75,25.98
  Bottom 0.508: v30.43,20.19 30.78,20.54 30.78,20.91 30.29,20.91 30.26,20.94 | 33.82,27.78 33.47,27.78 v33,28.25 | v33,28.25 33.07,28.32 v33.82,28.32 | v33,28.25 33.3,27.95 33.3,26.85 32.87,26.42 32.19,26.42 | 31.75,25.98 32.19,26.42 | 30.78,25.03 30.78,25.78 | 32.19,26.42 31.42,26.42 30.78,25.78 | 30.78,25.78 30.26,25.26 30.26,21.2 | 30.26,21.2 30.26,21.09 | 30.78,21.54 30.44,21.2 30.26,21.2
  Bottom 0.6: IC2.1 19.59,18.52 C29.2 19.59,20.71 C28.2 19.97,21.09 20,21.06 29.57,21.06 v30.43,20.19 30.48,20.14 v30.48,19.4
  Bottom 0.61: 30.78,20.91 30.78,21.54 30.78,25.03 30.8,25.03 v31.63,25.86 | v33.82,28.32 33.82,27.78 33.82,26.59 33.12,25.89 31.66,25.89
  pour Bottom (no thermals): 30,21.06 29.52,20.58 29.52,19.09 29.81,18.8 30.89,18.8 31.03,18.94 31.03,24.42 31.76,25.15 33.61,25.15 34.43,25.97 34.43,28.32 34.04,28.71 33.22,28.71 32.82,28.31 32.82,27.07 32.83,27.06 32.49,26.72 31.47,26.72 30,25.25 30,21.07 29.99,21.06
  pour Top (no thermals): 30.27,20.53 31.93,20.53 32.27,20.19 32.58,19.88 32.58,18.62 32.58,17.64 33.03,17.19 33.85,17.19 34.45,16.59 34.45,15.52 34.24,15.31 34.23,15.3 32.95,15.3 32.86,15.39 32.86,16.11 32.86,16.29 32.66,16.49 32.59,16.56 31.57,16.56 30.93,17.2 28.68,17.2 28.61,17.2 28.34,17.47 28.34,18 28.48,18.14 28.71,18.37 30.35,18.37 31.16,18.37 31.42,18.63 31.42,18.83 31.32,18.93 31.26,18.99 30.32,18.99 29.91,19.4 29.91,19.62 29.91,20.4 30.04,20.53 30.26,20.53
A0  (via drill 0.3 pad 0.6)
  Top 0.203: U5.38 25.06,31.85 25.63,32.42 26.31,32.42 26.78,31.95 26.78,31.09 26.79,31.08 26.79,30.67 27.58,29.88 27.58,27.96 27.76,27.78 v27.76,27.7
  Bottom 0.203: v27.76,27.7 27.09,27.03 27.09,26.06 26.65,25.62 23.95,25.62 22.21,27.36 R25.2 21.42,27.05 21.41,27.05 20.84,26.48 R26.1
A0_IN
  Bottom 0.203: 25.18,24.72 J7.1 24.2,24.7 22.42,26.48 R25.1
A1  (via drill 0.3)
  Top 0.203: U5.39 24.88,32.25 25.56,32.93 27.03,32.93 28.25,34.15 28.25,36.15 27.73,36.67 27.73,38.64 27.58,38.79 27.43,38.79 v27.29,38.93
  Bottom 0.203: v27.29,38.93 27.18,39.04 27.18,39.67 26.56,40.29 23.14,40.29 22.52,40.91 22.51,40.91 R20.2 R24.1
A1_IN
  Bottom 0.203: R20.1 23.23,39.3 J1.1
A2
  Top 0.203: U5.40 24.71,32.65
BOOT
  Top 0.203: R3.1 10.64,42.29 8.9,42.29 8.19,43 8.19,43.57 7.62,44.14 3.69,44.14 3.12,43.58 1.27,41.72 1.27,39.93 SW1.2
CHRG
  Top 0.203: D4.- 23.32,38.11 23.32,40.56 22.69,41.19 22.69,44.27 22.26,44.7 20.97,44.7 20.24,45.43 14.43,45.43 13.57,44.57 3.59,44.57 0.69,41.66 0.69,24.16 1.48,23.36 4.33,23.36 4.61,23.08 6.59,23.08 7.54,24.02 IC1.7
D0/TX0
  Top 0.203: U5.2 16.47,33.05 15.98,32.56 14.78,32.56 14.65,32.56 13.48,31.39 13.48,30.43 13.13,30.08 11.93,30.08 10.18,28.33 10.18,21.09 9.79,20.7 6.88,20.7 6.19,20 R12.1
D1/RX0  (via drill 0.3 pad 0.6)
  Top 0.203: R11.1 6.2,18.84 6.96,18.08 v7.98,18.08 | v8.08,20.01 8.21,20.14 10.04,20.14 10.57,20.67 10.57,28.03 12.18,29.64 13.29,29.64 13.84,30.18 13.84,31.11 14.93,32.21 16.21,32.21 16.65,32.65 U5.3
  Bottom 0.203: v8.08,20.01 8.08,18.18 v7.98,18.08
D2  (via drill 0.3 pad 0.6)
  Top 0.203: v18.27,32.39 18.13,32.25 U5.4
  Bottom 0.203: 17.98,32.39 v18.27,32.39 17.97,32.39 16.4,33.96 R38.1 16.21,33.81 Q3.2
D2_H
  Bottom 0.203: J9.1 11.01,45.3 11.68,44.63 11.68,38.63 12.8,37.51 R39.1 13.23,34.93 Q3.3
D3  (via drill 0.3 pad 0.6)
  Top 0.203: v14.49,30.79 15.55,31.85 U5.5
  Bottom 0.203: v14.49,30.79 15.34,31.64 Q9.2 15.67,31.82 R22.1
D3_H
  Bottom 0.203: J8.1 11.63,30.7 12.8,31.87 R19.1 12.92,31.88 13.31,32.27 Q9.3
D4/SDA0  (via drill 0.3 pad 0.6)
  Top 0.203: U5.6 16.08,31.45 13.75,29.12 12.28,29.12 10.95,27.79 10.95,20.69 12.32,19.32 12.32,17.42 11.66,16.76 11.66,15.53 13.29,13.9 13.29,9.68 v13.4,9.57
  Bottom 0.203: v13.4,9.57 14.82,9.57 15.21,9.18 15.21,8.61 15.58,8.24 Q12.2 16.71,8.24 R44.1
D4/SDA0_H
  Bottom 0.203: J11.2 10.61,14.1 12.4,12.31 12.4,11.02 12.77,10.65 12.77,9.34 13.23,8.88 Q12.3 14.69,8.44 R45.1
D5/SCL0  (via drill 0.3 pad 0.6)
  Top 0.203: U5.7 16.19,31.05 13.87,28.73 12.43,28.73 11.37,27.67 11.37,20.83 12.79,19.41 12.79,17.3 12.06,16.57 12.06,15.64 13.65,14.05 13.65,10.63 v14.1,10.18
  Bottom 0.203: v14.1,10.18 15.75,10.18 Q13.2 16.71,10.45 R46.1
D5/SCL0_H
  Bottom 0.203: Q13.3 13.77,11.09 13.7,11.02 13.69,11.02 R47.1 13.32,10.7 12.78,11.24 12.78,12.47 11.59,13.66 11.59,15.12 10.61,16.1 J11.1
D6
  Top 0.203: U5.8 16.41,30.65 14.1,28.34 12.6,28.34 11.81,27.54 11.81,20.94 13.29,19.46 13.29,17.27 12.49,16.47 12.49,15.78 14.09,14.18 14.09,11.17 14.84,10.42 14.84,9.85 13.84,8.85 13.84,7.84 13.45,7.45 12.84,7.45 11.94,6.55 10.43,6.55 9.49,5.61 8.15,5.61 7.45,4.91 7.45,2.97 8.53,1.88 J3.3
D7
  Top 0.203: U5.9 16.65,30.25 14.32,27.92 12.77,27.92 12.24,27.39 12.24,21.16 13.67,19.72 13.67,17.15 12.89,16.37 12.89,15.92 13.19,15.62 13.2,15.62 14.45,14.37 14.45,11.39 15.2,10.64 15.2,9.7 14.2,8.7 14.2,7.69 13.6,7.09 13.04,7.09 12.14,6.19 10.58,6.19 9.64,5.26 9.48,5.26 J3.4
D8/TX1  (via drill 0.3 pad 0.6)
  Top 0.203: U5.11 16.47,29.45 13.88,26.86 13.88,20.02 14.03,19.87 14.03,16.96 13.53,16.46 v13.53,16.14
  Bottom 0.203: v13.53,16.14 14.54,16.14 14.89,15.79 14.89,14.25 15.32,13.82 17.8,13.82 18.52,13.1 18.52,11.58 R40.1 19.18,11.53 Q10.2
D8/TX1_H
  Bottom 0.203: J10.2 24.31,12.1 23.3,11.09 Q10.3 21.14,12.23 R41.1
D9/RX1  (via drill 0.3 pad 0.6)
  Top 0.203: U5.12 16.57,29.05 14.39,26.86 14.39,15.71 v14.19,15.52
  Bottom 0.203: v14.19,15.52 14.19,13.9 14.69,13.4 17.69,13.4 18.16,12.93 18.16,12.12 17.9,11.86 17.9,9.91 R42.1 18.67,9.52 Q11.2
D9/RX1_H
  Bottom 0.203: R43.1 21.14,7.67 Q11.3 21.14,9.66 21.58,10.1 J10.1
D10
  Top 0.203: U5.13 16.68,28.65 14.8,26.77 14.8,11.59 16.14,10.25 16.14,8.71 14.09,6.66 13.11,6.66 12.23,5.78 10.78,5.78 9.99,4.98 9.99,3.07 J3.5
D11
  Top 0.203: U5.14 16.82,28.25 15.19,26.62 15.19,11.75 16.62,10.32 16.62,8.58 14.3,6.26 13.27,6.26 11.43,4.42 J3.6
D12
  Top 0.203: U5.15 17.77,27.11 16.48,27.11 15.58,26.21 15.58,11.92 17.03,10.47 17.03,8.38 14.55,5.9 13.48,5.9 12.49,4.91 12.49,3.11 J3.7
D13
  Top 0.203: U5.16 18.47,26.94 18.24,26.71 16.64,26.71 15.96,26.03 15.96,12.08 17.41,10.63 17.41,8.17 13.72,4.48 J3.8
D14
  Top 0.203: U5.17 18.87,26.82 18.4,26.35 16.86,26.35 16.36,25.85 16.36,12.28 17.83,10.81 17.83,8 15.07,5.23 15.07,3.07 J3.9
D15
  Top 0.203: U5.18 19.27,26.72 18.54,25.99 17.14,25.99 16.8,25.65 16.8,12.38 18.29,10.89 18.29,7.85 16.26,5.82 J3.10
D16
  Top 0.203: U5.27 22.87,26.93 23.55,26.26 23.55,22.87 19.7,19.02 19.7,6.26 19.1,5.66 18.11,5.66 17.61,5.16 17.61,2.91 18.63,1.88 J3.11
D17
  Top 0.203: U5.28 23.27,27.07 23.93,26.41 23.93,22.73 20.13,18.93 20.13,6.05 18.8,4.72 J3.12
D18
  Top 0.203: J3.13 20.09,3.13 20.09,5.25 20.54,5.71 20.54,18.84 24.37,22.67 24.37,27.99 U5.29
D19
  Top 0.203: J3.14 20.98,4.78 20.98,18.77 24.85,22.64 24.85,28.38 24.58,28.65 U5.30
D20
  Top 0.203: U5.31 24.84,29.05 25.23,28.66 25.23,22.49 21.35,18.61 21.35,6.2 22.62,4.93 22.62,2.91 23.65,1.88 J3.15
D21
  Top 0.203: U5.32 24.94,29.45 25.66,28.74 25.66,22.33 21.76,18.43 21.76,6.44 23.78,4.42 J3.16
D22
  Top 0.203: U5.34 24.77,30.25 26.07,28.95 26.07,22.2 22.18,18.31 22.18,6.85 23.2,5.83 24.61,5.83 25.21,5.22 25.21,3 26.33,1.88 J3.17
D23
  Top 0.203: U5.35 25.02,30.66 26.43,29.25 26.43,22.05 22.57,18.19 22.57,7.03 23.33,6.27 25.34,6.27 26.42,5.19 J3.18
D24
  Top 0.203: U5.36 25.2,31.05 26.79,29.46 26.79,6.61 27.7,5.7 27.7,3.14 J3.19
D25  (via drill 0.3 pad 0.6)
  Top 0.203: U5.37 25.44,31.45 25.57,31.32 | 25.57,31.32 27.15,29.74 27.15,7.08 28.96,5.27 J3.20 | v25.87,31.77 25.87,31.62 25.57,31.32 | v25.79,33.54 27.13,33.54 27.89,34.3 27.89,36 27.13,36.77 27.13,38.05 v27.11,38.07 | v25.99,36.56 25.47,37.08 D1.-
  Bottom 0.203: v25.87,31.77 25.87,33.46 v25.79,33.54 | v27.11,38.07 25.99,36.95 v25.99,36.56
DN
  Top 0.203: R5.1 20.49,38.81 20.01,39.3 19.71,39.3 18.25,40.76 J5.B7 18.25,42.97 18.12,43.1 17.37,43.1 17.25,42.98 J5.A7
DP
  Top 0.203: R6.1 19.59,38.89 17.76,40.72 17.74,40.72 | 17.74,40.72 J5.A6 | J5.B6 16.75,40.86 16.89,40.72 17.74,40.72
GND  (via drill 0.3, 0.3 pad 0.6, 0.35)
  Top 0.203: IC1.PAD 6.53,27.95 6.53,28.3 v6.53,28.53 | v18.24,28.36 18.64,28.36 18.82,28.18 19.58,28.18 19.67,28.09 U5.19 19.67,26.26 v19.32,25.91 | v17.66,25.31 17.16,24.81 17.16,22.54 v17.6,22.1
  Top 0.305: J5.A12 13.18,42.94 13.18,43.16 | 13.18,43.16 J5.P$2 | J5.B1 13.25,43.16 13.18,43.16 | J5.B12 21.77,43.18 | 21.77,43.18 J5.P$1 | J5.A1 21.77,42.88 21.77,43.18
  Top 0.5: R21.2 33.14,12.45 33.06,12.53 U1.2
  Top 0.508: C11.1 18.53,38.69 v18,39.22 | C13.1 21.48,38.86 v21.05,39.29 | v27.94,46.32 27.58,46.68 26.01,46.68 25.85,46.84 J4.P$4 22.07,47.6 J5.P$3 J5.P$4 9.39,47.36 J6.P$3 7.42,47.6 v7.32,47.7 6.23,46.61 v4.65,46.61 3.44,46.61 J6.P$4 | J4.P$2 28.17,41.93 28.16,41.94 27.99,42.11 | C19.1 5.87,13.8 v5.23,13.16 | IC1.6 v6.26,26 | v6.26,26 6.26,27.05 6.79,27.58 IC1.PAD 7.75,28.43 v7.75,28.45 8.8,29.5 IC1.1 9.09,30.66 9.5,30.66 v10.77,31.93 10.95,32.11 v10.95,33.85 | v1.8,27.38 C30.1 3.38,28.51 C31.1 | C31.1 3.4,27.71 v3.13,27.44 3.13,26.75 C32.1 3.28,26.36 v2.46,26.36 | IC1.3 6.26,28.8 v6.53,28.53 | J4.P$3 32.03,47.08 v30.76,47.08 | SW2.1 33.89,35.98 v33.89,36.45 | U2.2 32.79,24.66 32.33,24.2 32.33,22.11 32.82,21.62 v32.82,20.64 | 7.43,27.81 v7.43,25.96 6.3,25.96 v6.26,26 | C31.1 6.3,28.53 6.53,28.3 | v21.54,21.94 21.74,21.94 v22.37,22.57 22.64,22.84 C4.1 | v21.54,21.94 20.7,21.94 v20.67,21.91 18.91,21.91 v18.9,21.89 17.81,21.89 v17.6,22.1 | v19.32,25.91 19.1,25.69 X1.4 18.79,24.43 C3.1 17.66,24.55 v17.66,25.31 | X1.2 21.54,22.8 v21.54,21.94
  Top 0.6: U4.17 9.84,10.26 v7.3,10.26 | ANT1.P$1 4.84,10.43 v4.9,10.37 | ANT1.P$2 4.89,7.67 v4.91,7.69 | C22.1 33.62,18.15 C2.1 32.82,20.33 v32.82,20.64 | U1.2 33.02,13.35 v33.02,14.31 | v32.09,14.54 32.79,14.54 v33.02,14.31 | v33.02,14.31 33.98,14.31 v34.01,14.34 | v29.77,6.37 29.77,7.83 C33.1 31.22,7.92 C25.1 31.42,6.45 v31.05,6.08
  Top 0.61: 4.8,39.76 5.51,39.05 5.52,39.05 R9.2 | J6.P$2 4.01,42.69 v3.5,42.69 | J6.P$2 4.51,41.61 v3.48,41.61 | J6.P$2 3.66,40.76 v3.66,40.63 | U6.4 8.4,35.87 v8.4,35.14 | R15.1 9.98,32.72 v10.77,31.93 | v10.03,38.11 11.11,39.19 v12.82,39.19 | C14.1 28.18,32.96 27.76,32.54 27.76,31.71 v27.39,31.34 | v30.49,32.49 30.58,32.4 C20.1 31.89,32.04 C21.1 31.64,30.96 30.55,30.96 R37.1 30.5,31.52 v30.35,31.67 | v31.26,28.26 31.1,28.1 C24.1 | C24.1 30.26,26.58 C23.1 30.34,25.6 31.73,24.2 32.33,24.2 | v30.86,29.09 30.26,28.49 C24.1 | U4.1 v25.51,7.9 v25.5,7.89 | IC1.6 v6.26,23.75 | v8.17,22.39 7.79,22.01 4.46,22.01 3.38,20.93 v0.95,20.93 | SW1.1 2.1,36.6 J9.SS2 | J4.P$2 27.68,41.38 v27.25,41.38 27.15,41.28 | R36.2 26.45,41.28 27.15,41.28 | 27.15,41.28 27.23,41.28 v27.23,40.6 27.37,40.74 28.05,40.74 28.16,40.85 28.16,41.94
  Top 0.8: 28.17,41.93 v28.17,44.23
  Top 1.016: 4.8,39.76 J6.P$2
  Bottom 0.203: R24.2 21.3,39.54 v21.05,39.29
  Bottom 0.305: R8.1 20.29,39.91 20.98,39.22
  Bottom 0.406: 20.42,42.09 R8.1
  Bottom 0.5: 29.38,24.42 29.38,21.88
  Bottom 0.508: C6.1 19.77,31.72 v19.72,31.77 | C9.1 20.16,30.59 v19.77,30.98 | v28.17,44.23 28.17,46.09 v27.94,46.32 30,46.32 v30.76,47.08 31.48,47.8 J1.SS2 32.7,38.93 32.76,38.87 32.76,36.6 32.7,36.54 | v10.95,33.85 10.8,33.85 9.51,35.14 v8.4,35.14 8.4,36.48 v10.03,38.11 | v12.82,39.19 12.43,39.58 12.43,42.44 J5.P$2 | R7.2 15.09,41.9 15.09,41.67 17.54,39.22 v18,39.22 | v18,39.22 20.98,39.22 v21.05,39.29 21.99,38.35 | 19.64,37.59 19.9,37.32 C12.1 C7.1 21.99,38.35 | 19.64,37.59 v18,39.22 | v33.89,36.45 33.54,36.8 J1.SS1 32.7,36.54 | 32.7,36.54 J7.SS2 31.99,32.49 v30.49,32.49 30.35,32.35 v30.35,31.67 30.35,30.88 30.6,30.63 30.6,29.35 v30.86,29.09 30.86,28.66 v31.26,28.26 v31.27,28.25 v32.04,28.25 29.38,25.59 29.38,24.42 | v32.82,20.64 32.7,20.76 J7.SS1 | J10.SS2 32.7,19.48 | 1.03,20.93 v0.95,20.93 | 1.03,20.93 1.03,19.87 J11.SS1 2.3,15.3 4.44,13.16 v5.23,13.16 5.23,10.7 v4.9,10.37 6,10.37 v6.07,10.3 7.26,10.3 7.46,10.1 | J11.SS2 2.3,7.55 | 2.3,7.55 2.3,5.56 v1.52,4.78 2.01,4.29 3.69,4.29 J3.1 | J12.1 12.8,27.03 10.47,24.7 J8.4 8.69,24.7 v7.43,25.96 | v7.32,47.7 7.23,47.79 v4.21,47.79 v4.2,47.8 J9.SS1 3.5,46.6 v3.5,42.69 3.5,41.63 v3.48,41.61 3.66,41.43 v3.66,40.63 2.3,39.27 J9.SS2 J8.SS1 2.3,27.88 v1.8,27.38 2.46,26.72 v2.46,26.36 | C9.1 C10.1 20.54,29.58 v19.53,29.58 19.53,29.34 18.68,28.48 18.36,28.48 v18.24,28.36 19.41,28.36 20.41,27.36 R26.2 | C9.1 C6.1 | C6.1 C8.1 19.87,32.74 v19.75,32.62 19.75,34.48 18.35,35.88 18.35,36.3 19.64,37.59 | 21.99,38.35 23.63,38.35 23.98,38 C1.1 24.21,37.33 24.69,36.85 24.69,36.74 25.84,35.59 26.88,35.59 27.09,35.38 | 27.09,35.38 27.39,35.08 27.39,32.43 27.39,31.31
  Bottom 0.508: 27.09,35.38 29.01,37.3 29.01,39.03 27.44,40.6 v27.23,40.6 | v3.13,27.44 2.46,26.77 v2.46,26.36 | v2.46,26.36 2.46,26.22 v1.6,25.36 1.6,24.65 v2.2,24.05 2.3,23.95 J8.SS2 1.03,20.93 | v7.84,7.9 v7.83,7.91 v6.3,7.91 6.08,7.69 v4.91,7.69 4.77,7.55 2.3,7.55 | v9.36,7.91 11.07,7.91 v11.57,8.41 | v11.57,8.41 9.88,10.1 J11.4 | v25.5,7.89 27.02,6.37 26.42,5.77 18.24,5.77 17.95,5.47 17.11,5.47 16.68,5.9 13.77,5.9 12.57,7.1 12.57,7.41 v11.57,8.41 | J10.SS1 32.7,5.39 v32.76,5.33 | C28.1 17.95,21.75 v17.6,22.1
  Bottom 0.6: J11.4 7.46,10.1 v7.3,10.26 | J10.4 23.2,16.1 | 23.2,16.1 22.96,16.1 21.97,15.11 19.52,15.11 18.84,15.79 v18.84,16.99 | IC2.2 v18.85,17 v18.84,16.99 | C18.1 22.36,16.94 23.2,16.1 | v18.84,16.99 v18.83,17 v18.83,17.9 v18.82,17.91 18.82,18.27 18.07,19.03 C29.1 17.95,19.36 C28.1 16.7,19.6 C26.1 14.42,19.6 C27.1 | 27.02,6.37 27.16,6.51 v28.79,6.51
  Bottom 0.61: J9.4 10.03,39.07 v10.03,38.11 | R8.1 20.73,42.09 J5.P$1 | R7.2 14.29,42.06 J5.P$2 | v6.26,23.75 6.81,23.75 v8.17,22.39 | 27.37,32.45 27.39,32.43 | C34.1 C5.1 18.51,31.14 19.09,31.72 19.77,31.72 | v12.82,39.19 13.36,39.73 C17.1 C15.1 13.17,39.19 v12.82,39.19
  Bottom 0.813: J5.P$1 23.11,44.46 23.64,44.46 24.48,45.3 J1.4
  Bottom 1.016: J7.4 26.78,30.7 27.39,31.31 v27.39,31.34
  other vias: 2.3,36.8 4.42,1.13 3.83,3.76 30.75,1.11 33.88,4.1 33.92,6.34 27.69,32.55 33.74,40.58 31.43,44.29 33.74,44.77 31.03,48.76 23.57,48.82 15.55,48.9 6.43,48.84 1.16,44.86 1.03,22.8 8.7,23.19 2.52,18.31 1.27,14.19 1.32,10.45 3.34,14.1 24.37,7.01 24.14,7.87 2.82,11.42 4.16,11.41 4.03,6.6 3.14,5.79 18.83,15.93 33.63,20.61 34.05,21.26 34.04,9.55 34.06,8.19
  pour Bottom (rank 2, no thermals): -3.41,23.61 -3.41,48.16 -0.54,51.03 1.09,52.66 10.08,52.66 34.66,52.66 36.06,51.26 36.45,50.87 36.45,-1.09 34.12,-3.42 24.28,-3.42 0,-3.42 -0.93,-2.49 -3.41,-0.01 -3.41,23.57
  pour Top (rank 2, no thermals): -3.89,11.3 -3.89,48.58 0.71,53.18 34.82,53.18 37.17,50.83 37.17,-2.21 35.08,-4.3 -0.91,-4.3 -0.93,-4.28 -3.89,-1.32 -3.89,11.28
IO2
  Top 0.203: U4.15 8.83,12.87 7.84,13.86 7.84,16.62 6.14,18.32 3.67,18.32 2.49,19.5 SW3.1
N$1  (via drill 0.3 pad 0.6)
  Top 0.203: v24.28,34.87 24.28,34.82 23.75,34.29 U5.43
  Bottom 0.203: v24.28,34.87 24.28,36.13 C1.2 23.86,36.43 23.29,37 23.28,37 R1.2
N$2  (via drill 0.3 pad 0.6)
  Top 0.203: J5.B5 15.75,42.94 16.19,43.38 v16.67,43.38
  Bottom 0.203: v16.67,43.38 16.67,42.92 R7.1
N$3
  Top 0.61: U2.3 33.74,23.2 L1.1
  pour Top (no thermals): 33.47,26.95 33.47,27.19 33.71,27.43 34.26,27.43 34.41,27.28 34.41,22.48 34.17,22.24 33.99,22.06 33.48,22.06 33.08,22.46 33.08,22.61 33.08,24.58 33.08,24.91 33.27,25.1 33.48,25.31 33.48,26.94
N$4
  pour Top (no thermals): 32.2,13.77 32.17,13.8 28.38,13.8 27.71,13.13 27.71,11.97 27.71,10.98 27.91,10.78 28.75,10.78 28.97,11 28.99,11.02 28.99,11.99 29.71,12.71 29.86,12.71 29.94,12.79 32.09,12.79 32.28,12.98 32.28,13.06 32.28,13.71 32.19,13.8
N$5
  Top 0.203: U4.10 7.86,19.22 7.18,19.9 R12.2
N$6  (via drill 0.3 pad 0.6)
  Top 0.203: J5.A5 18.75,43.05 v18.09,43.71
  Bottom 0.203: v18.09,43.71 18.09,43.4 R8.2
N$7
  Top 0.203: R14.2 7.1,16.84 5.98,17.96 3.4,17.96 2.1,16.67 SW3.2
N$8
  Top 0.9: U4.18 ANT1.P$3
N$9
  Top 0.203: R23.1 29.93,30.6 29.93,30.59 30.49,30.03 R37.2 30.85,30.03 31.53,29.35 U2.5
N$10
  Top 0.203: R15.2 8.65,31.83 7.54,30.71 IC1.2
N$11
  Top 0.305: R18.1 24.05,38.96 D4.+
N$13
  Top 0.3: R16.2 34.01,11.96 R21.1 34.02,13.29 U1.3
N$14
  Top 0.305: R17.1 25.47,39.55 D1.+
QSPI_CS
  Top 0.203: U5.56 17.67,34.69 14.88,34.69 13.48,36.09 10.71,36.09 9.11,34.49 7.73,34.49 7.12,35.1 7.12,38.9 8.03,39.8 U6.1 9.93,41.2 R4.2 10.68,41.43 11.26,42.01 11.26,42.02 R3.2
QSPI_D0
  Top 0.203: U6.5 18.41,35.99 19.27,35.13 U5.53
QSPI_D1
  Top 0.203: U5.55 18.47,34.79 18.21,35.04 15.15,35.04 13.57,36.63 7.77,36.63 7.48,36.92 7.48,38.1 7.95,38.57 8.49,38.57 U6.2
QSPI_D2
  Top 0.203: U5.54 18.87,35 18.45,35.42 15.28,35.42 13.53,37.17 8.62,37.17 U6.3
QSPI_D3
  Top 0.203: U5.51 20.07,35.34 18.69,36.72 18.09,36.72 17.76,37.04 17.76,38.05 17.27,38.53 U6.7
QSPI_SCK
  Top 0.203: U6.6 16.93,37.27 17.84,36.36 18.54,36.36 19.67,35.23 U5.52
RESET  (via drill 0.3 pad 0.6)
  Top 0.203: U5.26 22.47,25.56 v22.54,25.49 | R13.2 29.48,32.91 C14.2 29.88,32.96 v30.35,33.43 | v31.45,39.28 31.8,38.93 33.57,38.93 33.4,39.1 SW2.2
  Bottom 0.203: v31.45,39.28 31.02,38.85 31.02,34.74 30.34,34.06 v30.34,33.44 v30.35,33.43 29.74,32.82 29.74,30.77 30.09,30.42 30.09,28.3 29.23,27.44 29.23,26.99 28.44,26.2 28.44,24.85 27.39,23.8 23.62,23.8 23.44,23.98 23.44,24.89 22.84,25.49 v22.54,25.49
RF_3V3  (via drill 0.3, 0.3 pad 0.6)
  Top 0.508: 25.97,19.36 25.83,19.22 U4.9 | U4.9 24.39,19.22 23.14,17.97 23.14,15.12 v23.25,15.01 | v6.24,16.72 6.21,16.7 R14.1 6.21,14.81 R10.1 | U4.9 25.51,19.93 v25.78,20.2
  Bottom 0.5: 10.14,17.29 10.21,17.22 12.54,17.22 13.11,17.79 C27.2 14.13,17.06 14.54,16.65 14.74,16.65 15.4,15.99 15.4,14.62 15.65,14.37 22.61,14.37 v23.25,15.01
  Bottom 0.508: v6.24,16.72 6.69,17.17 10.26,17.17 10.14,17.29 10.14,18.93 11.96,20.75 11.96,24.66 12.7,25.4 12.72,25.4 J12.2 | v25.78,20.2 23.92,20.2 C18.2
  Bottom 0.6: C26.2 15.94,17.93 | C26.2 14.16,17.82 C27.2 | IC2.5 15.96,17.95 C26.2
RF_RX  (via drill 0.3 pad 0.6)
  Top 0.203: U4.12 10.78,16.68 11.66,17.56 v11.66,18.02
  Bottom 0.203: v11.66,18.02 11.66,18.33 13.84,20.51 13.84,23.73 J12.3
RF_TX  (via drill 0.3 pad 0.6)
  Top 0.203: v11.46,19.04 11.46,18.81 10.6,17.95 U4.11 9.29,17.95 8.49,18.75 7.23,18.75 R11.2
  Bottom 0.203: v11.46,19.04 12.94,20.52 12.94,23.08 J12.4
RST
  Top 0.203: U4.16 8.17,11.6 7.14,12.63 C19.2 7.11,13.82 R10.2
USB_D+
  Top 0.203: U5.47 21.67,35.59 20.18,37.08 20.16,37.08 19.92,37.33 R6.2
USB_D-
  Top 0.203: U5.46 22.07,35.74 20.49,37.32 R5.2
XIN
  Top 0.203: U5.20 20.07,24.01 X1.1 18.61,23.53 C3.2
XOUT
  Top 0.203: U5.21 20.47,25.44 21.17,24.74 X1.3 22.33,24.74 C4.2

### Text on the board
tPlace: - | + | - | + | GND | RA-3V | RA-RX | RA-TX | 7 | 23 | 25 | 24
bPlace: www.elecrow.com | Lora RA-08H Node Board V1.0 | GP2 | GND | NC | 5V | NC | 5V | GND | A1 | GND | GP3 | NC | 5V | 5V | GND | NC | A0 | SCL-GP5 | TX1-GP8 | SDA-GP4 | RX1-GP9 | GND | SCL | SDA | 5V | 5V | TX1 | GND | RX1 | 11 | 7 | 3V3 | 25 | G | 24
